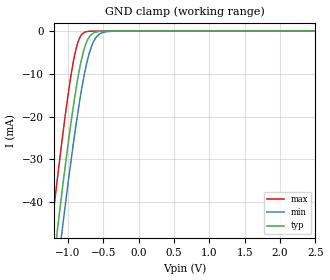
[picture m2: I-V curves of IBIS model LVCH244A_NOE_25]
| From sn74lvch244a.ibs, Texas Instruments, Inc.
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[Model]   LVCH244A_NOE_25
Model_type  Input
Vinl=0.7
Vinh=1.7
| variable   typ   min   max
C_comp   3.40pF   3.05pF   4.04pF
[Temperature Range]   40   100   -40
| Ambient temperature   25   85   -40
[Voltage range]   2.5   2.3   2.7
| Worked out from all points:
|   GND clamp passes 1 mA (typ) near -0.68 V on its own axis
[GND Clamp]
| LVCH244A_NOE_25
|   Voltage   I(typ)   I(min)   I(max)
-5.5V     -731.8mA   -738.6mA   -723.7mA
-1.25V    -60.73mA   -70.05mA   -48.77mA
-1.22V    -56.44mA   -65.77mA   -44.44mA
-1.145V   -45.9mA    -55.24mA   -33.86mA
-1.1V     -39.74mA   -49.06mA   -27.74mA
-1.075V   -36.38mA   -45.67mA   -24.43mA
-970mV    -22.98mA   -31.99mA   -11.73mA
-865mV    -11.47mA   -19.59mA   -2.924mA
-735mV    -2.503mA   -7.547mA   -134.2uA
-650mV    -566.3uA   -2.886mA   -13.44uA
-565mV    -106.5uA   -838.9uA   -1.322uA
2.5V      1.115nA    59.61nA    7.066pA
